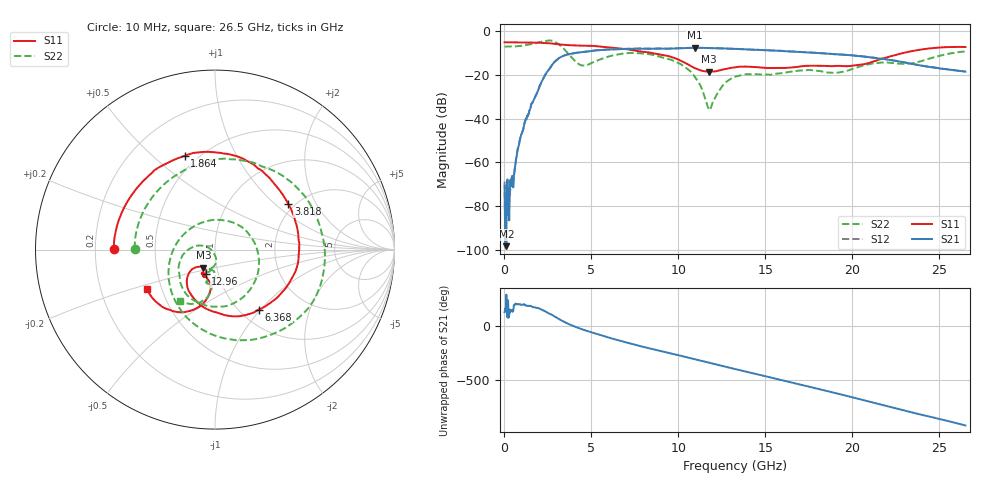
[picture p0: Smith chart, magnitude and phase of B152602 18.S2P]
!  2-Port S-parameters saved by WinCal
! VAR MeasName=S-Parameters (CALIBRATED_DATA) read from VNA (N5242A)
! VAR MeasDate=2016-1-5 16:27:57
! VAR NAME=B152602 18
! VAR FILENAME=B152602 18.S2P
! VAR DATE=2016-1-5 16:27:57
! VAR PHYS_PORTS=1,2
# Hz S DB R 50
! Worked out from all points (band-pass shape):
!   801 points, 10 MHz to 26.5 GHz, reference 50 ohm
!   highest |S21| = -7.51 dB at 10.94 GHz (marker M1); lowest = -98.4 dB at 109.3 MHz (marker M2)
!   |S21| within 3 dB of the highest: 3.664 GHz to 19.08 GHz (15.42 GHz wide, 136 % of centre)
!   lowest |S11| = -18.5 dB at 11.73 GHz (marker M3), VSWR 1.27, Z = 43.1 - j8.75 ohm
!   |S11| at or under -10 dB: 8.564 GHz to 22.88 GHz (14.31 GHz wide, 91 % of centre)
!   |S22| runs from -36.0 to -4.1 dB; largest |S21 - S12| = 0.0033
!   S11 on the Smith chart (normalised r, x): 10 MHz: 0.28, +0.00; 1.864 GHz: 0.43, +0.64; 3.818 GHz: 1.86, +1.23; 6.368 GHz: 1.22, -0.98; 12.96 GHz: 0.87, -0.24; 26.5 GHz: 0.41, -0.22
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1e7  -4.98 179.6  -70.72 126.4  -68.81 -168.8  -6.98 179.4
1.093375e8  -4.97 175.7  -98.43 -71.5  -84.95 15.8  -6.96 173.4
3.742375e8  -5.02 165.3  -70.99 139.5  -70.70 153.4  -6.92 157.0
1.102712e9  -5.15 137.7  -43.96 -162.6  -43.94 -162.9  -6.48 111.2
1.8643e9  -5.21 108.0  -28.33 165.1  -28.33 165.0  -5.31 55.4
2.493438e9  -5.39 82.0  -18.17 119.0  -18.17 119.0  -4.23 -4.5
2.990125e9  -5.83 61.7  -13.18 75.4  -13.18 75.4  -5.18 -64.4
3.420588e9  -6.18 45.7  -11.10 36.8  -11.10 36.9  -8.01 -116.3
3.817938e9  -6.35 31.8  -10.23 7.0  -10.24 7.0  -11.51 -163.4
4.447075e9  -6.55 9.4  -9.50 -32.1  -9.49 -32.0  -15.58 113.8
6.3676e9  -7.64 -53.5  -8.18 -126.9  -8.15 -126.8  -10.81 -42.4
7.592762e9  -8.92 -85.3  -7.91 -179.5  -7.88 -179.5  -9.96 -93.0
8.851038e9  -10.40 -111.2  -7.90 130.3  -7.85 130.2  -11.41 -135.3
1.093712e10  -16.80 -136.9  -7.51 49.8  -7.51 49.9  -20.75 165.7
1.173182e10  -18.46 -123.0  -7.64 18.2  -7.62 18.2  -35.29 -160.5
1.295699e10  -16.78 -111.2  -7.93 -29.4  -7.90 -29.3  -22.03 -87.6
1.3255e10  -16.47 -112.2  -8.01 -40.7  -7.99 -40.9  -20.82 -92.9
1.507619e10  -16.77 -118.5  -8.62 -110.3  -8.64 -110.5  -19.71 -106.1
1.769208e10  -15.71 -114.1  -9.74 148.7  -9.71 148.8  -17.79 -108.4
1.951326e10  -15.91 -111.0  -10.68 77.2  -10.67 77.3  -18.48 -94.0
2.209604e10  -11.64 -98.1  -12.99 -28.6  -12.92 -28.8  -14.32 -103.9
2.65e10  -7.15 -150.0  -18.42 157.0  -18.42 156.7  -9.21 -124.6
